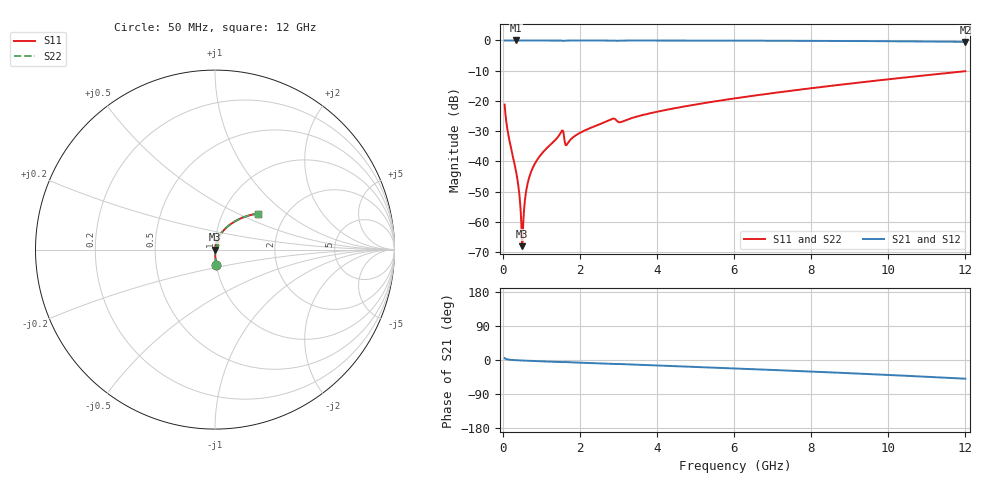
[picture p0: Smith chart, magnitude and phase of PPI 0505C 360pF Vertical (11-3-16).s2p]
# GHz S MA R 50
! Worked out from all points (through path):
!   1601 points, 50 MHz to 12 GHz, reference 50 ohm
!   highest |S21| = 0.00 dB at 341.3 MHz (marker M1); lowest = -0.5 dB at 12 GHz (marker M2)
!   group delay of S21, straight-line fit = 11.4 ps
!   lowest |S11| = -68.0 dB at 505.6 MHz (marker M3), VSWR 1.00, Z = 50 - j0.00819 ohm
!   |S11| at or under -10 dB: start of sweep to end of sweep
!   |S22| runs from -68.0 to -10.2 dB; largest |S21 - S12| = 0
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0.05  0.08714 -85.0  0.996 4.9  0.996 4.9  0.08714 -85.0
0.1620312  0.02448 -88.4  0.9994 1.0  0.9994 1.0  0.02448 -88.4
0.3412812  0.007118 -87.8  0.9996 -0.5  0.9996 -0.5  0.007118 -87.8
0.4085  0.003843 -85.5  0.9996 -0.9  0.9996 -0.9  0.003843 -85.5
0.46825  0.001466 -76.2  0.9996 -1.2  0.9996 -1.2  0.001466 -76.2
0.5055937  0.0003973 -11.9  0.9996 -1.4  0.9996 -1.4  0.0003973 -11.9
0.5429375  0.001243 69.7  0.9996 -1.5  0.9996 -1.5  0.001243 69.7
0.6026875  0.003053 80.4  0.9995 -1.8  0.9995 -1.8  0.003053 80.4
0.6699063  0.004959 82.9  0.9995 -2.1  0.9995 -2.1  0.004959 82.9
0.767  0.007512 84.0  0.9995 -2.5  0.9995 -2.5  0.007512 84.0
0.9089063  0.01099 84.3  0.9994 -3.1  0.9994 -3.1  0.01099 84.3
1.513875  0.0305 73.6  0.9938 -5.8  0.9938 -5.8  0.0305 73.6
1.551219  0.03255 62.5  0.9875 -5.9  0.9875 -5.9  0.03255 62.5
1.670719  0.01922 70.7  0.9952 -5.5  0.9952 -5.5  0.01922 70.7
2.044156  0.03061 80.9  0.9984 -7.2  0.9984 -7.2  0.03061 80.9
2.828375  0.05027 73.7  0.9934 -10.4  0.9934 -10.4  0.05027 73.7
3.059906  0.0446 71.9  0.9931 -10.7  0.9931 -10.7  0.0446 71.9
4.038312  0.06699 74.4  0.9963 -14.6  0.9963 -14.6  0.06699 74.4
6.025  0.1104 67.0  0.9923 -22.3  0.9923 -22.3  0.1104 67.0
8.019156  0.1628 58.9  0.9847 -30.6  0.9847 -30.6  0.1628 58.9
10.01331  0.2284 50.1  0.9712 -39.5  0.9712 -39.5  0.2284 50.1
12  0.3104 40.2  0.9477 -49.4  0.9477 -49.4  0.3104 40.2
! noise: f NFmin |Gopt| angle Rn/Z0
0.05  0.0003104  0.8329  0.2181  0.0003919
1.372  0.003996  0.6747  3.573  0.002367
2.701  0.007721  0.6699  7.01  0.00448
4.031  0.007106  0.5154  9.881  0.002542
5.36  0.008337  0.4693  12.62  0.00263
6.682  0.009851  0.45  15.25  0.002945
8.012  0.01149  0.4413  17.8  0.003342
9.341  0.01326  0.4401  20.27  0.003823
10.67  0.01521  0.4453  22.68  0.004412
12  0.01739  0.4563  25.09  0.005146
